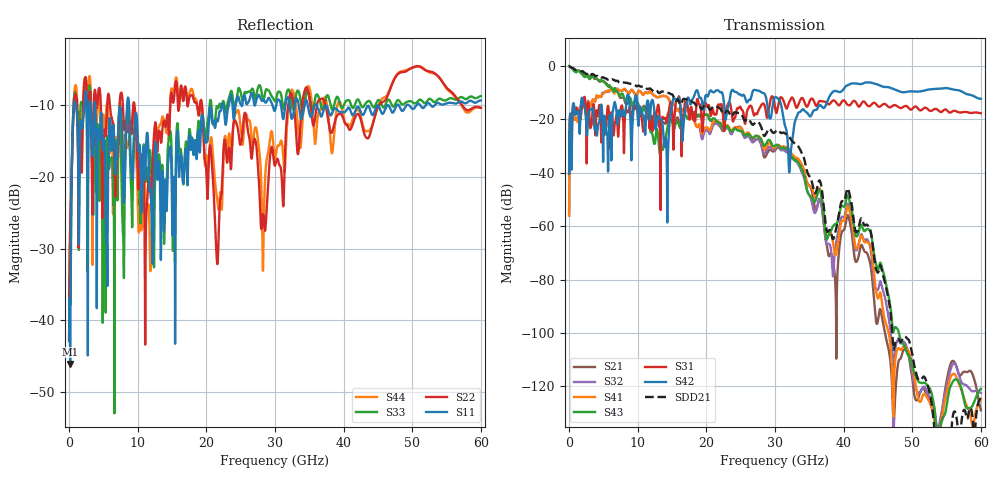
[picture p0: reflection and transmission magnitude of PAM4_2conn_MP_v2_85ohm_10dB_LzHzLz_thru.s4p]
! Info: Touchstone file created by Circ.  Input file=FAB50GbE_2conn_Midplane_Examax_Topo2_v2_85ohm_10dB_LzHzLz.circ
# Hz S RI R 50
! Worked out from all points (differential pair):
!   6000 points, 10 MHz to 60 GHz, reference 50 ohm
!   strongest paths, dB at 10 MHz, 15.01 GHz, 30.01 GHz, 45.01 GHz, 60 GHz:
!     S42: -40.3, -14.5, -11.7, -7.0, -12.3
!     S31: -40.4, -17.2, -15.4, -15.1, -17.7
!     S43: -0.1, -20.9, -29.8, -76.2, -120.9
!     S41: -56.1, -13.9, -30.4, -87.1, -124.8
!     S32: -56.1, -14.1, -30.9, -83.8, -122.5
!     S21: -0.1, -18.3, -31.5, -95.2, -128.9
!   taken as a pair (ports 3,1 in; 4,2 out), SDD21 dB: -0.1, -10.7, -24.7, -77.4, -124.5
!   lowest |S11| = -46.1 dB at 160 MHz (marker M1), VSWR 1.01, Z = 50.3 + j0.381 ohm
!   |S11| at or under -10 dB: 3.814 GHz to 8.456 GHz (4.641 GHz wide, 75.7 % of centre); 8.744 GHz to 22.28 GHz (13.53 GHz wide, 87.3 % of centre); 36.07 GHz to 46.34 GHz (10.27 GHz wide, 24.9 % of centre)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
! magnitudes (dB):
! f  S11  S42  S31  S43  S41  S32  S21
! 10 MHz  -42.8  -40.3  -40.4  -0.1  -56.1  -56.1  -0.1
! 160 MHz  -46.1  -18.2  -18.1  -0.4  -31.6  -31.7  -0.4
! 900 MHz  -9.6  -18.1  -17.4  -2.2  -20.1  -20.1  -1.9
! 14.01 GHz  -20.4  -27.3  -19.4  -27.6  -11.2  -11.3  -21.7
! 32 GHz  -9.2  -36.2  -14.0  -31.9  -30.9  -33.0  -32.0
! 38.84 GHz  -10.4  -9.4  -13.4  -59.2  -70.8  -67.1  -84.6
! 60 GHz  -9.3  -12.3  -17.7  -120.9  -124.8  -122.5  -128.9
